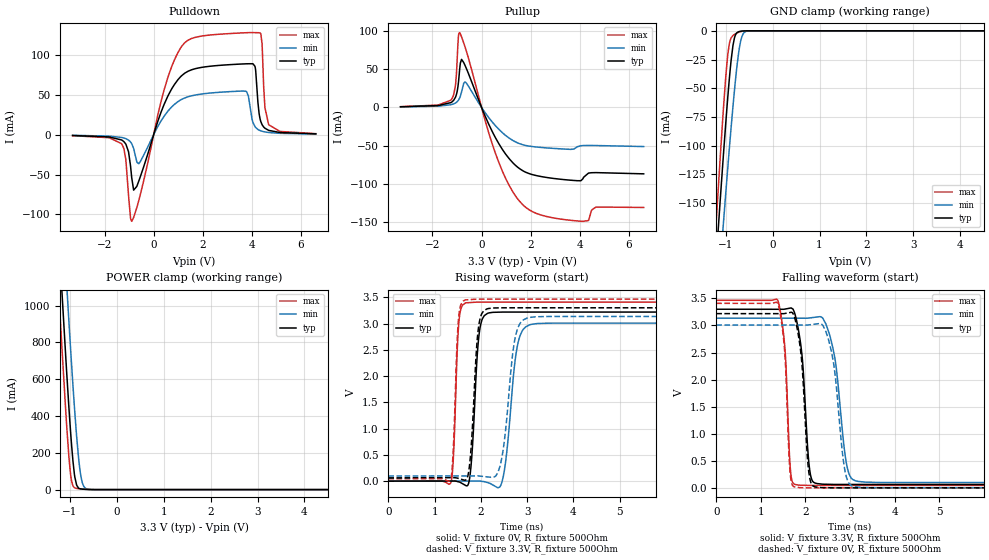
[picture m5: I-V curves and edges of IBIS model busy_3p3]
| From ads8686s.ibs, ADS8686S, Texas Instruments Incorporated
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|   busy_3p3 Model
[Model]   busy_3p3
Model_type   3-state
Polarity   Non-Inverting
Vmeas = 1.65
Vref = 1.65
Cref = 15pF
Rref = 50
|   typ   min   max
C_comp   1.51pF   1.51pF   1.55pF
[Voltage Range]   3.3   3.135   3.465
[Temperature Range]   27   125   -40
[Pullup Reference]   3.3   3.135   3.465
[Pulldown Reference]   0   0   0
[Power Clamp Reference]   3.3   3.135   3.465
[GND Clamp Reference]   0   0   0
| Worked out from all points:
|   slope of the pulldown table from 0 to 0.495 V, typ, clamps not added: 11.6 ohm
|   slope of the pullup table from 0 to 0.495 V, typ, clamps not added: 14 ohm
|   GND clamp passes 1 mA (typ) near -0.73 V on its own axis
|   POWER clamp passes 1 mA (typ) near -0.64 V on its own axis
|   falling waveform, V_fixture 3.3V, R_fixture 500Ohm: 20-80 % time 158ps typ, 245ps min, 117ps max; typ from 3.3 V to 0.063 V
|   rising waveform, V_fixture 0V, R_fixture 500Ohm: 20-80 % time 120ps typ, 192ps min, 83.7ps max; typ from 0 V to 3.22 V
|   rising waveform, V_fixture 3.3V, R_fixture 500Ohm: 20-80 % time 123ps typ, 205ps min, 83.6ps max; typ from 0.063 V to 3.3 V
|   falling waveform, V_fixture 0V, R_fixture 500Ohm: 20-80 % time 152ps typ, 228ps min, 114ps max; typ from 3.22 V to 0 V
[Pulldown]
|   Voltage   I(typ)   I(min)   I(max)
-3.3V     -1.063mA   -777.2uA   -1.275mA
-1.3V     -6.763mA   -3.55mA    -11.64mA
-894.3mV  -53.73mA   -11.28mA   -108.6mA
-597.3mV  -57.46mA   -36.13mA   -81.6mA
412.5mV   36.94mA    22.52mA    54.65mA
1.096V    72.59mA    43.51mA    108.6mA
3.759V    88.82mA    54.34mA    127.8mA
4.006V    88.91mA    19.21mA    128mA
4.363V    16.42mA    4.791mA    126.4mA
4.531V    8.045mA    3.437mA    33.87mA
4.689V    5.328mA    2.703mA    12.31mA
6.6V      1.008mA    739.3uA    1.25mA
[GND Clamp]
|   Voltage   I(typ)   I(min)   I(max)
-3.3V     -1.543A    -1.46A     -1.676A
-1.3V     -258.7mA   -305.1mA   -234mA
-1.201V   -198.3mA   -250.3mA   -166.4mA
-1.181V   -186.3mA   -239.5mA   -153.1mA
-1.112V   -145.1mA   -201.8mA   -107.6mA
-1.053V   -110.7mA   -170.1mA   -70.71mA
-953.7mV  -57.22mA   -118.6mA   -20.38mA
-844.8mV  -12.86mA   -65.95mA   -4.113mA
-726mV    -834uA     -19.91mA   -1.308mA
-636.9mV  -154.4uA   -3.384mA   -325.6uA
-488.4mV  -6.167uA   -57.71uA   -9.96uA
6.6V      0A         0A         0A
[Pullup]
|   Voltage   I(typ)   I(min)   I(max)
-3.3V     884.5uA    660.8uA    1.037mA
-1.241V   6.535mA    3.663mA    9.905mA
-1.063V   13.44mA    5.885mA    29.2mA
-943.8mV  32.22mA    9.475mA    92.8mA
-894.3mV  49.3mA     12.32mA    98.31mA
-815.1mV  63.09mA    20.41mA    92.68mA
-646.8mV  53.23mA    32.88mA    76.82mA
570.9mV   -40.05mA   -24.18mA   -60.78mA
1.68V     -83.09mA   -48.98mA   -127.8mA
4.046V    -96.11mA   -50.23mA   -149.4mA
4.66V     -85.52mA   -49.98mA   -130.7mA
6.6V      -87.13mA   -51.31mA   -131.3mA
[POWER Clamp]
|   Voltage   I(typ)   I(min)   I(max)
-3.3V     11.43A     11.88A     11.16A
-1.241V   1.403A     1.894A     1.097A
-1.171V   1.089A     1.579A     784.6mA
-1.063V   618.6mA    1.097A     329.3mA
-1.023V   459.5mA    927.8mA    189.3mA
-973.5mV  278mA      723.2mA    63.13mA
-894.3mV  69.04mA    420.6mA    9.281mA
-815.1mV  8.435mA    175.6mA    5.211mA
-765.6mV  3.51mA     75.42mA    3.892mA
-706.2mV  1.932mA    19.5mA     2.558mA
-617.1mV  815.2uA    2.229mA    1.058mA
6.6V      0A         0A         0A
[Ramp]
R_load = 500
|   typ   min   max
dV/dt_r   1.9313/1.19529e-10   1.80504/1.92021e-10   2.04523/8.36688e-11
dV/dt_f   1.94226/1.58392e-10   1.82241/2.43513e-10   2.05211/1.17458e-10
[Falling Waveform]
V_fixture = 3.3V
V_fixture_min = 3.135V
V_fixture_max = 3.465V
R_fixture = 500Ohm
C_fixture = 0F
|   Time   V(typ)   V(min)   V(max)
0s        3.3V       3.135V     3.465V
1.38ns    3.299V     3.134V     3.464V
1.751ns   3.242V     3.134V     67.92mV
1.921ns   2.457V     3.134V     48.29mV
2.094ns   332.4mV    3.139V     44.96mV
2.213ns   89.68mV    3.152V     44.95mV
2.612ns   63.78mV    2.593V     44.95mV
2.917ns   63.27mV    455.4mV    44.94mV
3.113ns   63.26mV    132.1mV    44.94mV
10ns      62.9mV     97.65mV    44.81mV
[Rising Waveform]
V_fixture = 0V
V_fixture_min = 0V
V_fixture_max = 0V
R_fixture = 500Ohm
C_fixture = 0F
|   Time   V(typ)   V(min)   V(max)
0s        -85.86nV   -10.09nV   -60.23nV
1.344ns   2.656mV    1.735mV    -39.4mV
1.52ns    -13.53mV   1.962mV    2.984V
1.668ns   -80.8mV    2.152mV    3.392V
1.969ns   2.849V     2.542mV    3.409V
2.144ns   3.194V     -26.83mV   3.409V
2.457ns   3.218V     -13.71mV   3.409V
2.783ns   3.219V     2.548V     3.409V
3.055ns   3.219V     2.976V     3.409V
10ns      3.219V     3.008V     3.409V
[Rising Waveform]
V_fixture = 3.3V
V_fixture_min = 3.135V
V_fixture_max = 3.465V
R_fixture = 500Ohm
C_fixture = 0F
|   Time   V(typ)   V(min)   V(max)
0s        62.9mV     97.65mV    44.81mV
1.344ns   65.51mV    99.22mV    33.59mV
1.508ns   54.05mV    99.41mV    2.994V
1.654ns   17.32mV    99.58mV    3.447V
1.945ns   2.903V     99.14mV    3.465V
2.127ns   3.277V     82.08mV    3.465V
2.409ns   3.299V     269.8mV    3.465V
2.722ns   3.3V       2.641V     3.465V
2.998ns   3.3V       3.104V     3.465V
10ns      3.3V       3.135V     3.465V
[Falling Waveform]
|Gnd
V_fixture = 0V
V_fixture_min = 0V
V_fixture_max = 0V
R_fixture = 500Ohm
C_fixture = 0F
|   Time   V(typ)   V(min)   V(max)
0s        3.219V     3.008V     3.409V
1.38ns    3.218V     3.008V     3.407V
1.737ns   3.188V     3.008V     23.73mV
1.909ns   2.393V     3.008V     3.021mV
2.075ns   288.2mV    3.011V     354.7uV
2.197ns   22.64mV    3.023V     104uV
2.531ns   1.992mV    2.693V     99.58uV
2.868ns   241uV      396.8mV    95.09uV
3.055ns   234.7uV    29.79mV    92.6uV
10ns      -2.68nV    -82.25nV   -36.56nV
